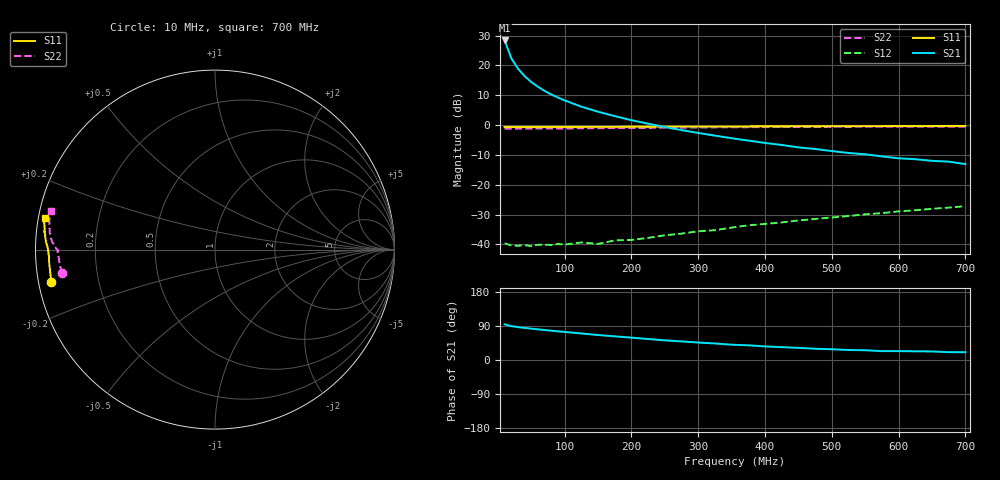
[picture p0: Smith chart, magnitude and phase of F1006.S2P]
! Date: Mon Aug 07 14:44:00 1995
# MHZ  S  MA  R  50.0000
!  POLYFET RF DEVICES
!  F1006
!  S PARAMETERS
!  VDS=28V, IDQ=1.20A
!FREQ  S11MAG S11ANG S21MAG S21ANG S12MAG S12ANG S22MAG S22ANG
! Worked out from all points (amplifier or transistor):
!   34 points, 10 MHz to 700 MHz, reference 50 ohm
!   highest |S21| = 28.4 dB at 10 MHz (marker M1)
!   |S21| within 3 dB of that: start of sweep to 15.05 MHz
!   unconditionally stable (mu >= 1): 178.9 MHz to 348.2 MHz
!   at 60 MHz: K = 0.44, MSG = 26.5 dB, |S12| = -40.1 dB
!   at 300 MHz: K = 1.09, MAG = 14.7 dB, |S12| = -35.6 dB
!   at 700 MHz: K = 0.72, MSG = 7.1 dB, |S12| = -27.2 dB
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10  0.9296 -168.9  26.17 94.1  0.01042 10.3  0.8644 -171.3
20  0.9264 -174.5  13.21 89.3  0.0096 9.0  0.8703 -175.7
30  0.9269 -176.4  8.819 86.9  0.00947 8.8  0.8719 -177.1
40  0.9253 -177.5  6.594 84.7  0.0097 11.5  0.8749 -178.0
50  0.926 -178.1  5.266 82.7  0.00933 14.2  0.8747 -178.5
60  0.9287 -178.6  4.368 80.9  0.00989 14.9  0.8764 -178.9
70  0.9271 -178.8  3.727 79.0  0.00986 16.0  0.8776 -179.3
80  0.9298 -179.5  3.253 77.3  0.00977 20.6  0.877 -179.3
90  0.9298 -179.6  2.883 75.6  0.01015 23.3  0.8744 -179.6
100  0.9274 -179.7  2.583 74.0  0.0099 21.8  0.8754 -179.8
125  0.9308 179.9  2.033 70.0  0.01079 28.8  0.8818 179.9
150  0.9328 179.3  1.67 65.9  0.01019 34.5  0.8852 179.6
175  0.9335 179.0  1.41 62.4  0.01165 38.0  0.8929 178.8
200  0.9377 178.5  1.205 59.0  0.01188 44.9  0.8944 178.4
250  0.9403 177.9  0.9261 51.8  0.01421 52.1  0.9033 177.8
300  0.9428 177.0  0.7369 46.1  0.01657 59.8  0.9135 176.5
350  0.947 176.1  0.6011 40.3  0.0191 59.8  0.9167 175.8
375  0.9479 175.8  0.5489 38.7  0.02087 63.4  0.9207 175.1
475  0.952 174.0  0.3967 29.8  0.02669 67.1  0.9318 172.5
600  0.9606 171.7  0.2771 23.5  0.03574 65.7  0.9379 169.3
675  0.9654 170.2  0.2438 20.6  0.0414 65.4  0.9415 167.1
700  0.9656 169.4  0.2214 20.6  0.04363 64.9  0.9392 166.7
